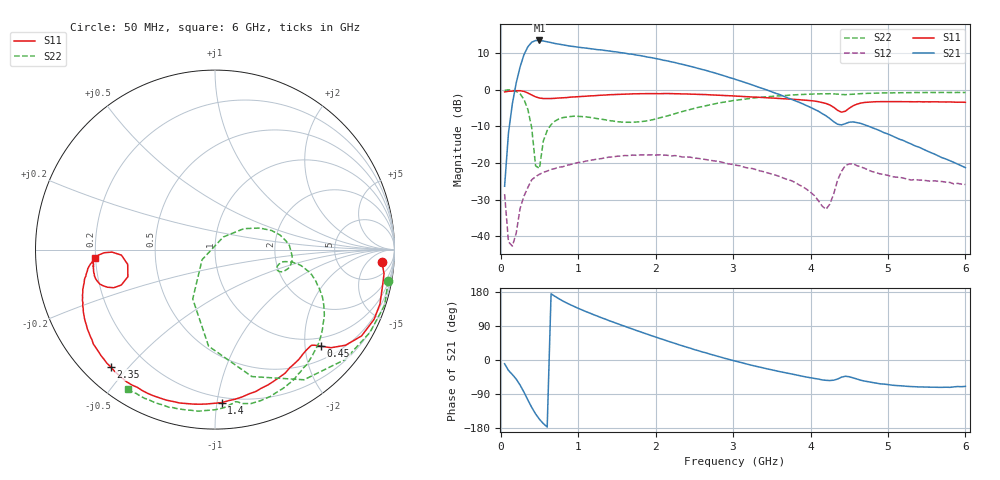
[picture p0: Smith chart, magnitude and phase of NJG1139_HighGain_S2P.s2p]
! Created Thu Jun 04 16:16:13 2009
# hz S ma R 50
! 2 Port Network Data from SP6.SP block
! freq  magS11  angS11  magS21  angS21  magS12  angS12  magS22  angS22
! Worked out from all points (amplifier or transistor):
!   120 points, 50 MHz to 6 GHz, reference 50 ohm
!   highest |S21| = 13.4 dB at 500 MHz (marker M1)
!   |S21| within 3 dB of that: 320.5 MHz to 1.439 GHz (1.119 GHz wide, 127 % of centre)
!   unconditionally stable (mu >= 1): start of sweep to 97.8 MHz; 102.8 MHz to 256.7 MHz; 2.67 GHz to end of sweep
!   at 1.05 GHz: K = 0.63, MSG = 15.6 dB, |S12| = -19.8 dB
!   at 3.05 GHz: K = 1.20, MAG = 9.0 dB, |S12| = -20.7 dB
!   at 6 GHz: K = 10.78, MAG = -11.0 dB, |S12| = -25.9 dB
!   lowest NFmin = 0.75 dB at 500 MHz
!   S11 on the Smith chart (normalised r, x): 50 MHz: 14, -14; 450 MHz: 0.79, -2.36; 1.4 GHz: 0.16, -1.03; 2.35 GHz: 0.08, -0.45; 6 GHz: 0.20, -0.03
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5e7  0.9323 -4.1  0.04802 -10.0  0.03754 168.0  0.9809 -10.2
1e8  0.9515 -8.1  0.2572 -27.5  0.008369 140.8  0.9945 -18.2
1.5e8  0.956 -13.0  0.6417 -38.3  0.007302 152.8  0.9787 -28.2
2.5e8  0.968 -23.7  2.047 -66.2  0.02389 157.5  0.8785 -55.7
3e8  0.9476 -30.5  3.005 -84.9  0.03519 144.8  0.7366 -73.8
3.5e8  0.9021 -36.2  3.852 -105.3  0.04613 130.6  0.5389 -93.8
4e8  0.8463 -40.2  4.445 -125.0  0.05888 115.8  0.3013 -114.3
4.5e8  0.7991 -42.3  4.69 -142.2  0.06493 101.5  0.09118 -142.0
5e8  0.7695 -43.8  4.7 -156.4  0.06998 90.8  0.08423 56.8
6e8  0.7562 -46.3  4.503 -177.0  0.07739 75.5  0.2775 25.6
7e8  0.7622 -50.4  4.272 168.0  0.08381 66.3  0.3723 12.5
8.5e8  0.7796 -57.8  4.011 150.7  0.09268 56.1  0.4227 -1.1
1.05e9  0.8091 -68.3  3.747 132.2  0.1027 45.3  0.4289 -11.7
1.4e9  0.8532 -87.5  3.378 103.7  0.12 28.4  0.3787 -18.9
2.05e9  0.8812 -119.4  2.603 57.0  0.1291 -1.0  0.412 -9.5
2.35e9  0.8742 -131.7  2.211 37.2  0.1203 -12.8  0.5051 -11.4
3.05e9  0.8153 -153.7  1.36 -3.9  0.09258 -34.9  0.7199 -32.6
4.05e9  0.6995 -173.3  0.5401 -48.6  0.03584 -41.5  0.8744 -69.4
4.2e9  0.6481 -177.4  0.44 -53.6  0.02329 -6.8  0.8794 -74.9
4.5e9  0.558 -159.3  0.3599 -44.1  0.09687 -4.4  0.8624 -83.2
5.05e9  0.6875 -169.1  0.2352 -66.4  0.06533 -40.1  0.9049 -98.2
6e9  0.6719 -175.9  0.08622 -69.6  0.05078 -50.3  0.9153 -122.1
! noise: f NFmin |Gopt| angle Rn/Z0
5e+07  1.393  0.7347  6.78  1.027
7e+08  0.8191  0.6056  59.67  0.2762
1.35e+09  0.88  0.6905  96.69  0.2397
2e+09  0.9798  0.7511  120.9  0.1935
2.65e+09  1.146  0.7815  137.8  0.1444
3.35e+09  1.461  0.7882  151.5  0.09725
4e+09  2.047  0.7684  162  0.06837
4.65e+09  3.314  0.715  171.2  0.07395
5.3e+09  6.154  0.6252  178.3  0.2041
6e+09  12.48  0.5305  -179.5  1.318
